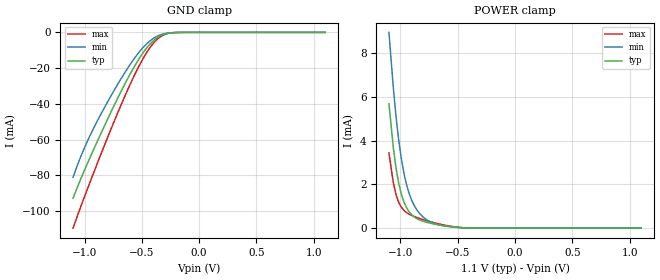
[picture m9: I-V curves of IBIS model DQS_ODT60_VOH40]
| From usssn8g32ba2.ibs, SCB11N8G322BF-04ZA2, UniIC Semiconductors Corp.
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|   Model DQS_ODT60_VOH40
[Model] DQS_ODT60_VOH40
Model_type Input
Vinl =  0.135V
Vinh =  0.305V
C_comp   1.020pF   1.010pF   1.030pF
[Model Spec]
Vinh   0.305V   0.297V   0.319V
Vinl   0.135V   0.127V   0.149V
[Add Submodel]
|  Submodel_name   Mode
ODT60_VOH40_DQDQS   Non-Driving
[Temperature Range]   25.000   0.105k   -40.000
[Voltage Range]   1.100V   1.060V   1.170V
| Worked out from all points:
|   GND clamp passes 1 mA (typ) near -0.30 V on its own axis
|   POWER clamp passes 1 mA (typ) near -0.95 V on its own axis
[GND_clamp]
|Voltage   I(typ)   I(min)   I(max)
-1.1V     -92.78mA   -81.05mA   -109.5mA
-1.031V   -81.73mA   -69.22mA   -97.17mA
-939mV    -68.18mA   -56.02mA   -81.64mA
-824mV    -52mA      -41.83mA   -62.83mA
-686mV    -33.62mA   -26.41mA   -41.32mA
-571mV    -19.76mA   -15.06mA   -24.85mA
-479mV    -10.5mA    -7.76mA    -13.5mA
-410mV    -5.313mA   -3.84mA    -6.916mA
-341mV    -2.007mA   -1.45mA    -2.59mA
-272mV    -506.9uA   -403.5uA   -609.8uA
-180mV    -45.65uA   -51.35uA   -43.55uA
1.1V      0A         0A         0A
[POWER_clamp]
|Voltage   I(typ)   I(min)   I(max)
-1.1V     5.691mA    8.967mA    3.44mA
-1.062V   3.709mA    6.444mA    2.092mA
-1.039V   2.781mA    5.152mA    1.546mA
-1.016V   2.086mA    4.085mA    1.193mA
-970mV    1.21mA     2.539mA    818.5uA
-947mV    943.7uA    2.005mA    716.7uA
-901mV    610.1uA    1.27mA     581.3uA
-855mV    430.7uA    824.1uA    484.6uA
-786mV    289.9uA    439.4uA    366uA
-671mV    155.9uA    155.9uA    203.6uA
-441mV    13.2uA     12.79uA    15.03uA
1.1V      0A         0A         0A
